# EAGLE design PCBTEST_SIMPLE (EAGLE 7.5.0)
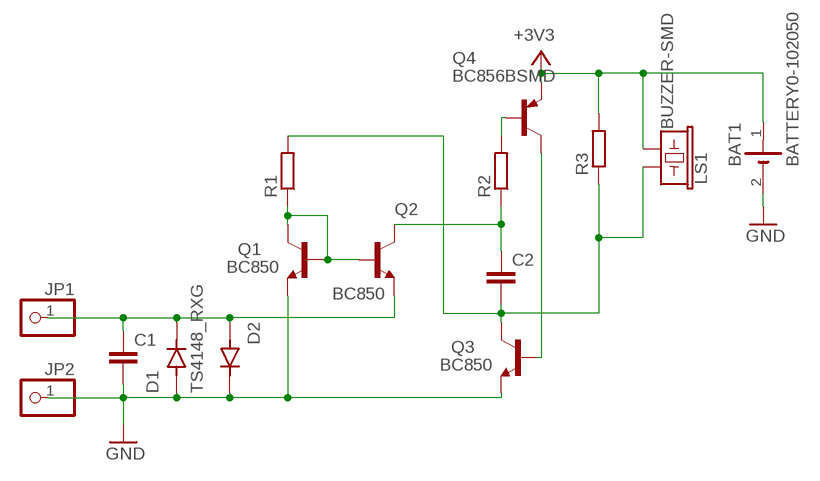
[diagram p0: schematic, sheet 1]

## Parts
BAT1  BATTERY0-102050  [BATTERY102050]
C1  C-EUC1206  [C1206]
C2  C-EUC1206  [C1206]
D1  TS4148_RXG  [DIO_TS4148_RXG]
D2  TS4148_RXG  [DIO_TS4148_RXG]
JP1  PINHD-1X1CB  [1X01-CLEANBIG]
JP2  PINHD-1X1CB  [1X01-CLEANBIG]
LS1  BUZZER-SMD  [BUZZER-CCV]
Q1  BC850  [SOT23]
Q2  BC850  [SOT23]
Q3  BC850  [SOT23]
Q4  BC856BSMD  [SOT23-BEC]
R1  R-EU_R1206  [R1206]
R2  R-EU_R1206  [R1206]
R3  R-EU_R1206  [R1206]

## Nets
+3V3: BAT1.1(+) LS1.- Q4.E R3.2
GND: BAT1.2(-) C1.2 D1.A D2.C(K) JP2.1 Q1.2(E) Q3.2(E)
N$3: C1.1 D1.C(K) D2.A JP1.1 Q2.2(E)
N$4: C2.2 LS1.+ Q3.3(C) R1.2 R3.1
N$5: C2.1 Q2.3(C) R2.1
N$6: Q1.1(B) Q1.3(C) Q2.1(B) R1.1
N$8: Q4.B R2.2
N$9: Q3.1(B) Q4.C

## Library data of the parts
BAT1 = battery:BATTERY0-102050
C1 C2 = rcl:C-EU: CAPACITOR, European symbol
D1 D2 = TS4148_RXG:TS4148_RXG: Check availability Check availability Check availability; AVAILABILITY: In Stock; CHECK_PRICES: https://www.snapeda.com/parts/TS4148%20RXG/Taiwan+Semiconductor/view-part/?ref=eda; DESCRIPTION: 1206 (Ceramics) 75V 0.15A Switching Diode & Array; MF: Taiwan Semiconductor; MP: TS4148 RXG; PACKAGE: 1206-2 Taiwan Semiconductor; PRICE: None; SNAPEDA_LINK: https://www.snapeda.com/parts/TS4148%20RXG/Taiwan+Semiconductor/view-part/?ref=snap
JP1 JP2 = adafruit:PINHD-1X1: Pin header 1x1 for 0.1" spacing
LS1 = SparkFun-Electromechanical:BUZZER: Buzzer; PROD_ID: COMP-08568
Q1-Q3 = transistor:BC850: NPN TRANSISTOR
Q4 = transistor-pnp:BC856*: PNP Transistror
R1-R3 = rcl:R-EU_: RESISTOR, European symbol

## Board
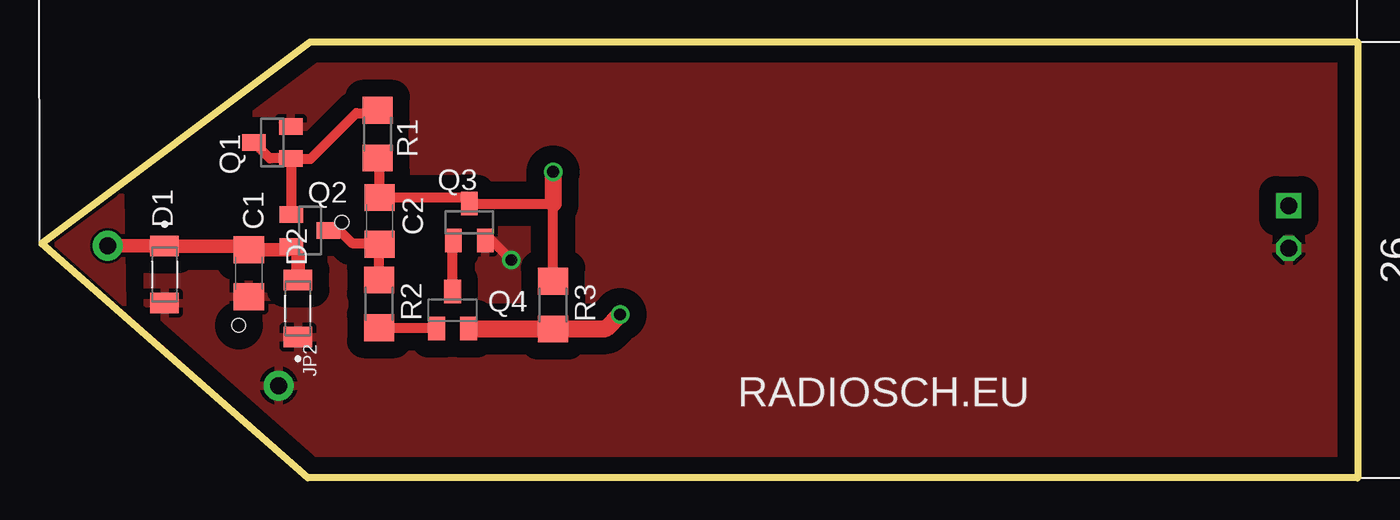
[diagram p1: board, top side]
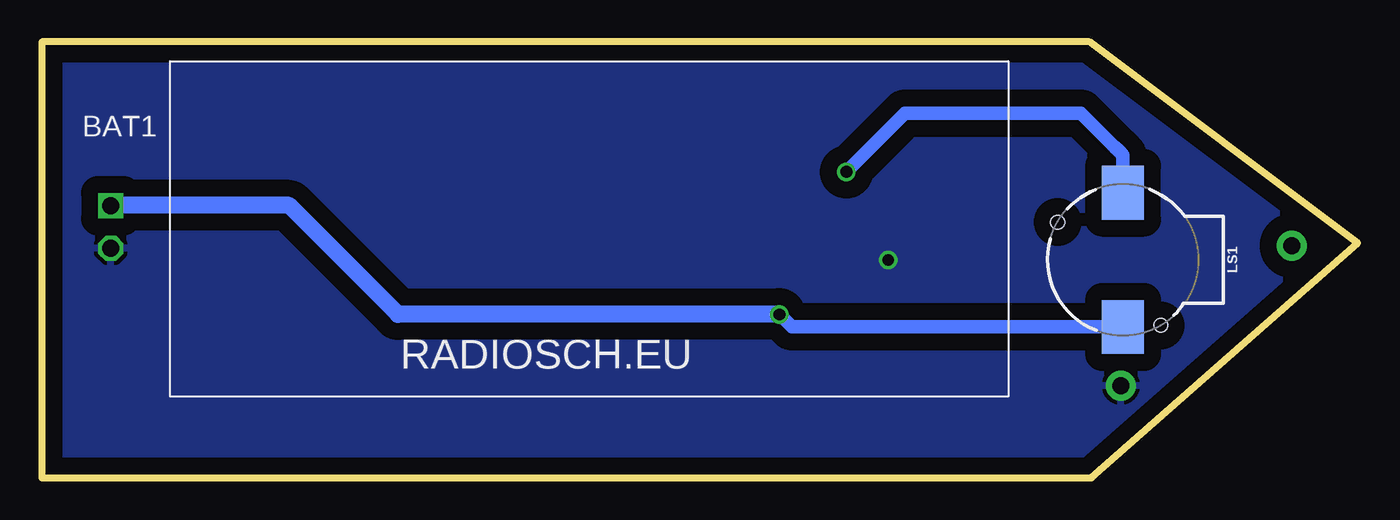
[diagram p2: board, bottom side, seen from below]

Size 78.5 x 26 mm. Coordinates in mm from the lower left corner, seen from the top.
Outline: 0,14 16,26 78.5,26 78.5,0 15.88,0 0,14
Copper layers (1*16): Top 0.035mm / dielectric 1.5mm / Bottom 0.035mm
Design rules "default *": minimum track width 10mil, minimum drill 20mil, track to track 6mil, track to pad 6mil, pad to pad 6mil, via to via 6mil, smd to smd 6mil, copper to edge 6mil, drill to drill 6mil, minimum pad ring 10mil, minimum via ring 8mil, stop-mask expansion 4mil, vias tented up to drill 20mil, thermal gap 10mil

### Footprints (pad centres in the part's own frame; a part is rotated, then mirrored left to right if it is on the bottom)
BATTERY102050 = drill 1 square: 1 -2.54,-7.62 | drill 1 octagon: 2 -2.54,-10.16
C1206 = smd 1.6 x 1.8: 1 -1.4,0; 2 1.4,0
DIO_TS4148_RXG = smd 1.2 x 1.7: A 1.7,0; C -1.7,0
1X01-CLEANBIG = drill 1.016 pad 1.778: 1 0,0
BUZZER-CCV = smd 3.2 x 2.5: + 4,0; - -4,0 | hole 0.8: -3.9,-2.25; 2.25,3.9
SOT23 = smd 1 x 1.4: 1 -0.95,-1.1; 2 0.95,-1.1; 3 0,1.1
SOT23-BEC = smd 1 x 1.4: B -0.95,-1.1; C 0,1.1; E 0.95,-1.1
R1206 = smd 1.6 x 1.803: 1 -1.422,0; 2 1.422,0

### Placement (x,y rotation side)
BAT1  71.85,23.85 0 bottom
C1  12.35,12.2 270 top
C2  20.15,15.32 90 top
D1  7.33,12.12 270 top
D2  15.28,10.1 90 top
JP1  3.93,13.85 0 top
JP2  14.12,5.5 0 top
LS1  14,13 90 bottom
Q1  13.75,20 90 top
Q2  16,14.75 270 top
Q3  25.5,15.25 0 top
Q4  24.5,10 0 top
R1  20.02,20.5 270 top
R2  20.12,10.38 270 top
R3  30.5,10.3 270 top

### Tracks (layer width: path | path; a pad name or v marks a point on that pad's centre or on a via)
+3V3  (via drill 0.7)
  Top 1.016: 30.48,8.9 33.65,8.9 v34.5,9.75 | Q4.E 30.48,8.9 | 30.48,8.9 R3.2
  Bottom 0.813: LS1.- 33.75,9 v34.5,9.75
  Bottom 1.016: v34.5,9.75 57.25,9.75 63.75,16.25 74.37,16.25 BAT1.1
GND  (via drill 0.7)
  Top 0.61: Q3.2 26.85,14.15 v28,13
  pour Top (isolate 1.016, rank 2): 0.5,14.25 16,24.75 78.75,25.5 79,0.5 16,-0.25
  pour Bottom (isolate 1.016): -0.12,13.88 16.12,25 77.62,25 77.88,0.88 58.88,0.88 16.38,1 0,13.88
N$1
  pour Top: 0.75,13.88 4.62,16.75 4.75,16.88 4.88,10.25
N$3
  Top 0.813: JP1.1 7.3,13.85 D1.C 12.12,13.82 C1.1 | 12.15,13.8 C1.1 | C1.1 14.7,13.6 Q2.2 15.28,13.43 D2.A
N$4  (via drill 0.7)
  Top 0.61: R3.1 30.5,16.35 Q3.3 25.12,16.73 C2.2 20.15,18.95 R1.2
  Top 1.016: v30.5,18.25 30.5,16.35
  Bottom 0.813: v30.5,18.25 27,21.75 16.5,21.75 14.5,19.75 14.25,19.5 14,19.25 LS1.+
N$5
  Top 0.61: Q2.3 17.75,14.75 18.5,14 20.07,14 C2.1 20.12,13.9 R2.1
N$6
  Top 0.61: Q2.1 14.9,19 14.88,19.02 | Q1.3 13.6,19.05 Q1.1 14.88,19.02 | 14.88,19.02 16.02,19.02 18.75,21.75 19.85,21.75 R1.1
N$8
  Top 0.61: R2.2 23.5,8.95 Q4.B
N$9
  Top 0.61: Q4.C 24.5,14.1 Q3.1

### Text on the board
tPlace: RADIOSCH.EU
bPlace: RADIOSCH.EU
